PROGRAM MAIN

VAR CONSTANT
	cInitSource			: ST_MA_MultiArray_InitPars := ( eTypeCode := eMA_TypeCode_LREAL, nDims := 1, aDimSizes := [cBufferLength]);
END_VAR

VAR
	(* Input *)
	nInputSelection		: UDINT := 1;						// Switch between hardware and function generator	
	nSample				: UDINT;   
	aEl3632 AT %I*		: ARRAY[1..cOversamples] OF INT;	// Input from hardware e.g. EL3632
	
	(* Signal Generator *)
	fbFunctionGenerator		: FB_FunctionGenerator;
	fbFunctionGeneratorExt	: FB_FunctionGenerator;
	
	(* Source buffers *)	
	aBuffer				: ARRAY[1..cOversamples] OF LREAL;								// local varibale -> to source
	aBufferExt			: ARRAY[1..cOversamples] OF LREAL;								// local varibale -> to source
	fbSource			: FB_CMA_Source :=(	stInitPars 		:= cInitSource,				// Initialize source buffers
											nOwnID 			:= eID_Source,
											aDestIDs		:= [eID_FFT, eID_ZoomFFT],
											nResultBuffers	:= 6);

	(* Result buffers *)										
	aFFTResult			: ARRAY[1..cFFTResult] OF LCOMPLEX;				// local result variable <- from sink
	aZoomFFTResult		: ARRAY[1..cZoomFFTResult] OF LCOMPLEX;			// local result variable <- from sink
    
	fbSink_FFT			: FB_CMA_Sink := (nOwnID := eID_SinkFFT);		// Initialize sink buffers
	fbSink_ZoomFFT		: FB_CMA_Sink := (nOwnID := eID_SinkZoomFFT);	// Initialize sink buffers
	
	(* post-processing of fft *)
	bCalculate1			: BOOL;											// true if fft calculation ready
	bCalculate2			: BOOL;											// true if zoom fft calculation ready	
	aSpectrumAbs        : ARRAY[1..cFFTResult] OF LREAL; 				// magnitude spectrum
	aZoomSpectrumAbs	: ARRAY[1..cZoomFFTResult] OF LREAL; 			// zoomed magnitude spectrum
	
	(* band *)
	fCenter				: LREAL := cSetFrequency;
	fLower				: LREAL := cLower;
	fUpper				: LREAL := cUpper;
	
	(* error monitoring *)
	fbErrHist	: FB_HRErrHist;
END_VAR

(* Input *) 
CASE nInputSelection OF
	0:  (* input from EL3632 *)
		FOR nSample := 1 TO cOversamples DO
			aBuffer[nSample] := INT_TO_LREAL(aEl3632[nSample]);
		END_FOR
	1:  (* signal generator *)		
		fbFunctionGenerator(	fFrequency 	:= cSetFrequency,
								fAmplitude 	:= cSetAmplitude,
								eFunction 	:= E_FunctionType.Sine,
								aSignal		:= aBuffer );
		fbFunctionGeneratorExt(	fFrequency 	:= cSetFrequencyExt,
								fAmplitude 	:= cSetAmplitude / 2,
								eFunction 	:= E_FunctionType.Sine,
								aSignal		:= aBufferExt );
        // add DC to signal
		FOR nSample := 1 TO cOversamples DO
			aBuffer[nSample] := cDC + aBuffer[nSample] + aBufferExt[nSample];
		END_FOR								
END_CASE					

(* Call source to collect data *)
fbSource.Input1DStd( pDataIn 		:= ADR(aBuffer),
				  	nDataInSize 	:= SIZEOF(aBuffer), 
				  	eElementType 	:= eMA_TypeCode_LREAL,
				  	nOptionPars		:= cCMA_Option_MarkInterruption );
IF fbSource.bError THEN
	fbErrHist.AddError(bErr:=TRUE, hrErrCode:=fbSource.hrErrorCode, sErrSource:='MAIN.fbSource'); // error monitoring
	// ToDo: if error
END_IF

(* Push results to sink *)
fbSink_FFT.Output1DStd(	pDataOut 		:= ADR(aFFTResult), 
						nDataOutSize 	:= SIZEOF(aFFTResult), 
						eElementType 	:= eMA_TypeCode_LCOMPLEX, 
						nOptionPars		:= 0,
						bNewResult		=> bCalculate1 );
IF fbSink_FFT.bError THEN
	fbErrHist.AddError(bErr:=TRUE, hrErrCode:=fbSink_FFT.hrErrorCode, sErrSource:='MAIN.fbSink_FFT'); // error monitoring
	// ToDo: if error
END_IF

fbSink_ZoomFFT.Output1DStd(	pDataOut 		:= ADR(aZoomFFTResult), 
							nDataOutSize 	:= SIZEOF(aZoomFFTResult), 
							eElementType 	:= eMA_TypeCode_LCOMPLEX, 
							nOptionPars		:= 0,
							bNewResult		=> bCalculate2 );
IF fbSink_ZoomFFT.bError THEN
	fbErrHist.AddError(bErr:=TRUE, hrErrCode:=fbSink_ZoomFFT.hrErrorCode, sErrSource:='MAIN.fbSink_ZoomFFT'); // error monitoring
	// ToDo: if error
END_IF

(* post-process fft result *)
IF bCalculate1 OR bCalculate2 THEN
	// Calculate absolute value as aFFTResult is of complex type
	FOR nSample := 1 TO cFFTResult DO			   	   
	   aSpectrumAbs[nSample] := SQRT(aFFTResult[nSample].re * aFFTResult[nSample].re + aFFTResult[nSample].im * aFFTResult[nSample].im);       
	   // scale spectrum
	   IF nSample = 1 THEN
		   aSpectrumAbs[nSample] := aSpectrumAbs[nSample] / cFFTLength;   // scale DC value
	   ELSE
		   aSpectrumAbs[nSample] := 2 * aSpectrumAbs[nSample] / cFFTLength; // scale frequencies not equal to 0
	   END_IF
	END_FOR;
	
	// Calculate absolute value as aZoomFFTResult is of complex type
	FOR nSample := 1 TO cZoomFFTResult DO			   	   
	   	aZoomSpectrumAbs[nSample] := SQRT(aZoomFFTResult[nSample].re * aZoomFFTResult[nSample].re + aZoomFFTResult[nSample].im * aZoomFFTResult[nSample].im);       
	   	// scale spectrum
		aZoomSpectrumAbs[nSample] := 2 * aZoomSpectrumAbs[nSample] / cFFTLength;
	END_FOR;
END_IF

END_PROGRAM
